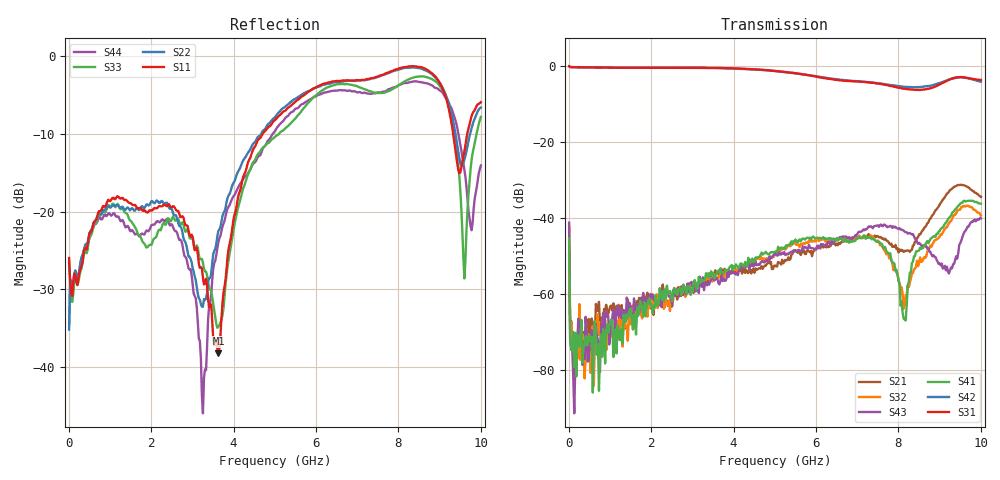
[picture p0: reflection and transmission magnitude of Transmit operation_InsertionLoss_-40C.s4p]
! Device:  ADRF5545A
! Description: Dual-Channel, Receiver Front End
! Frequency:  2.4 -  4.2 GHz
! Ports:
!	ANT-CHA	= Port 1
!	ANT-CHB	= Port 2
!  TXOUT-CHA = Port 3
!	TXOUT-CHB = Port 4
! VDD1-CHA, VDD1-CHB, VDD2-CHA, VDD2-CHB, and SWVDD-CHAB = 5 V
! SWCTRL-CHAB = 5 V,  PD-CHAB = 5 V,BP-CHA=BP-CHB=0V
! Temp=-40C
! Data:  Data was collected using a calibrated 4 port network analyzer and de-embedded using AtaiTec's In Situ De-Embedding.
! Note:  Analog Devices supplies this data as a sample of measured data
!  for this product.  Your particular data for this product may vary.
!  Data was taken at -40 degrees C.
!  Analog Devices reserves the right to change this data at anytime.
!Correction: S11(Full 4 Port(1,2,3,4))
!S12(Full 4 Port(1,2,3,4))
!S13(Full 4 Port(1,2,3,4))
!S14(Full 4 Port(1,2,3,4))
!S21(Full 4 Port(1,2,3,4))
!S22(Full 4 Port(1,2,3,4))
!S23(Full 4 Port(1,2,3,4))
!S24(Full 4 Port(1,2,3,4))
!S31(Full 4 Port(1,2,3,4))
!S32(Full 4 Port(1,2,3,4))
!S33(Full 4 Port(1,2,3,4))
!S34(Full 4 Port(1,2,3,4))
!S41(Full 4 Port(1,2,3,4))
!S42(Full 4 Port(1,2,3,4))
!S43(Full 4 Port(1,2,3,4))
!S44(Full 4 Port(1,2,3,4))
!S4P File: Measurements: <S11,S12,S13,S14>,
!<S21,S22,S23,S24>,
!<S31,S32,S33,S34>,
!<S41,S42,S43,S44>:
# Hz S  dB  R 50
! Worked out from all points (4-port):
!   401 points, 10 MHz to 10 GHz, reference 50 ohm
!   strongest paths, dB at 10 MHz, 2.507 GHz, 5.005 GHz, 7.503 GHz, 10 GHz:
!     S31: 0.0, -0.5, -1.3, -4.6, -3.6
!     S42: -0.1, -0.4, -1.3, -4.5, -4.1
!     S41: -45.4, -61.9, -49.0, -46.3, -36.2
!     S43: -41.2, -62.9, -49.6, -42.0, -40.1
!     S32: -41.8, -61.5, -49.3, -46.0, -39.3
!     S21: -50.0, -63.4, -52.6, -44.8, -34.5
!   lowest |S11| = -38.2 dB at 3.631 GHz (marker M1), VSWR 1.02, Z = 51.2 - j0.434 ohm
!   |S11| at or under -10 dB: start of sweep to 4.711 GHz; 9.326 GHz to 9.671 GHz (344.4 MHz wide, 3.63 % of centre)
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1e7  -25.96 -66.8  -40.36 -53.3  -0.08 -3.6  -47.39 -14.9
     -49.97 -146.8  -35.15 -107.9  -52.32 -101.6  0.05 -2.7
     -0.01 -3.6  -41.81 -151.2  -26.47 -44.9  -65.19 38.5
     -45.40 94.0  -0.09 -2.9  -41.24 105.2  -34.38 -86.0
2.098e8  -29.45 -80.7  -74.57 6.8  -0.32 -5.3  -83.15 -70.5
         -72.48 83.5  -28.70 -75.8  -76.81 104.2  -0.30 -5.0
         -0.32 -5.3  -76.49 -39.5  -29.37 -74.4  -73.96 91.1
         -70.80 -177.7  -0.29 -5.0  -71.86 122.0  -28.74 -80.0
3.631375e9  -38.19 -20.1  -53.65 55.2  -0.47 -92.4  -54.63 173.6
            -54.90 55.1  -22.48 16.7  -55.11 159.9  -0.50 -89.6
            -0.48 -92.4  -55.48 159.6  -34.70 -174.5  -55.40 -69.2
            -53.97 -176.0  -0.48 -89.5  -57.13 -77.2  -23.95 -32.8
4.6054e9  -10.74 31.2  -53.11 37.6  -0.91 -120.8  -50.52 142.9
          -53.32 39.5  -10.36 28.5  -50.51 128.4  -0.95 -117.2
          -0.92 -120.8  -50.32 129.5  -12.54 -100.7  -51.30 -144.1
          -50.38 147.2  -0.94 -117.2  -52.15 -137.4  -12.90 -91.9
8.15185e9  -1.47 35.9  -48.97 -55.8  -5.97 153.4  -65.08 135.8
           -48.68 -59.1  -1.56 26.4  -64.16 -14.2  -5.44 161.0
           -5.97 153.4  -62.60 -3.2  -3.29 72.6  -43.60 174.4
           -66.82 175.9  -5.44 161.2  -43.66 174.6  -3.51 100.5
9.6004e9  -12.28 157.8  -31.46 -166.6  -2.96 105.4  -35.72 -47.3
          -31.43 -166.8  -13.32 124.3  -36.94 -71.5  -3.05 113.9
          -2.97 105.4  -36.87 -71.1  -28.59 -46.3  -44.01 23.7
          -35.45 -48.3  -3.04 114.0  -43.67 22.2  -14.65 27.9
1e10  -5.97 174.2  -34.49 122.6  -3.62 78.5  -36.10 -117.7
      -34.45 123.0  -6.65 161.2  -39.08 -146.9  -4.09 88.9
      -3.62 78.5  -39.34 -145.3  -7.87 -129.0  -40.31 -55.1
      -36.24 -117.5  -4.09 89.1  -40.11 -55.5  -14.09 -92.8
